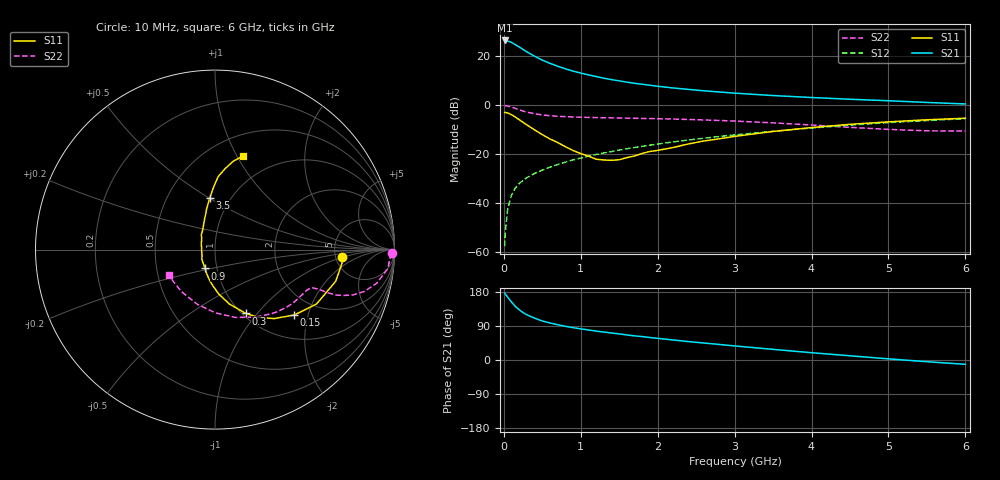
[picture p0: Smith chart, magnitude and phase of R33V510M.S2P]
! SIEMENS Small Signal Semiconductors
! BFR181
! Si NPN RF Bipolar Junction Transistor in SOT23
! VCE = 3.5 V  IC = 10 mA
! Common Emitter S-Parameters:  May  1996
# GHz  S  MA  R  50
!  f  S11  S21  S12  S22
! GHz  MAG  ANG  MAG  ANG  MAG  ANG  MAG  ANG
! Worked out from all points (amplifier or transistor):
!   36 points, 10 MHz to 6 GHz, reference 50 ohm
!   highest |S21| = 26.6 dB at 10 MHz (marker M1)
!   |S21| within 3 dB of that: start of sweep to 216.4 MHz
!   unconditionally stable (mu >= 1): 770.7 MHz to 2.659 GHz
!   at 250 MHz: K = 0.61, MSG = 26.8 dB, |S12| = -30.8 dB
!   at 1.4 GHz: K = 1.06, MAG = 13.2 dB, |S12| = -19.0 dB
!   at 6 GHz: K = 0.85, MSG = 3.0 dB, |S12| = -5.5 dB
!   S11 on the Smith chart (normalised r, x): 10 MHz: 5.75, -0.92; 150 MHz: 1.51, -1.64; 300 MHz: 1.04, -0.88; 900 MHz: 0.88, -0.19; 3.5 GHz: 0.80, +0.51; 6 GHz: 0.72, +1.06
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0.01  0.7103 -3.2  21.27 176.7  0.0013 91.9  0.9836 -1.2
0.02  0.7117 -6.1  21 173.8  0.0026 86.3  0.9774 -2.6
0.05  0.6954 -14.7  20.72 165.8  0.0075 79.5  0.9678 -6.4
0.1  0.6417 -28.2  19.4 153.0  0.0145 77.8  0.9197 -11.8
0.15  0.5726 -39.5  17.42 141.3  0.0203 72.8  0.863 -15.7
0.2  0.5063 -49.4  15.65 132.5  0.025 70.4  0.8085 -18.2
0.25  0.4465 -57.6  13.91 125.1  0.0288 68.6  0.7617 -19.6
0.3  0.3952 -64.2  12.38 119.3  0.033 68.5  0.7239 -20.5
0.4  0.3135 -75.2  10.11 110.5  0.0402 68.3  0.6709 -21.0
0.5  0.2498 -84.9  8.406 103.0  0.0469 69.1  0.6344 -20.9
0.6  0.2043 -92.9  7.22 97.7  0.054 69.1  0.6109 -21.0
0.7  0.172 -100.3  6.314 93.1  0.0613 69.9  0.5956 -21.2
0.9  0.1186 -117.7  5.01 85.3  0.0761 69.9  0.576 -21.8
1.1  0.0908 -144.0  4.194 79.3  0.0907 70.2  0.5641 -23.2
1.3  0.0757 -166.8  3.585 73.7  0.1055 69.8  0.5557 -24.8
1.6  0.0848 153.7  2.974 66.1  0.1288 68.9  0.5453 -27.9
2.2  0.1363 119.5  2.262 52.9  0.1775 65.6  0.5221 -35.8
2.8  0.2057 104.4  1.871 41.0  0.2295 61.3  0.489 -45.3
3.5  0.2909 95.6  1.581 28.1  0.2935 55.1  0.4365 -59.7
4.5  0.4072 87.5  1.329 11.1  0.392 44.2  0.3529 -89.4
5.5  0.5044 78.2  1.143 -4.5  0.4869 31.2  0.2998 -129.1
6  0.5429 73.4  1.064 -11.4  0.53 24.1  0.2955 -151.2
